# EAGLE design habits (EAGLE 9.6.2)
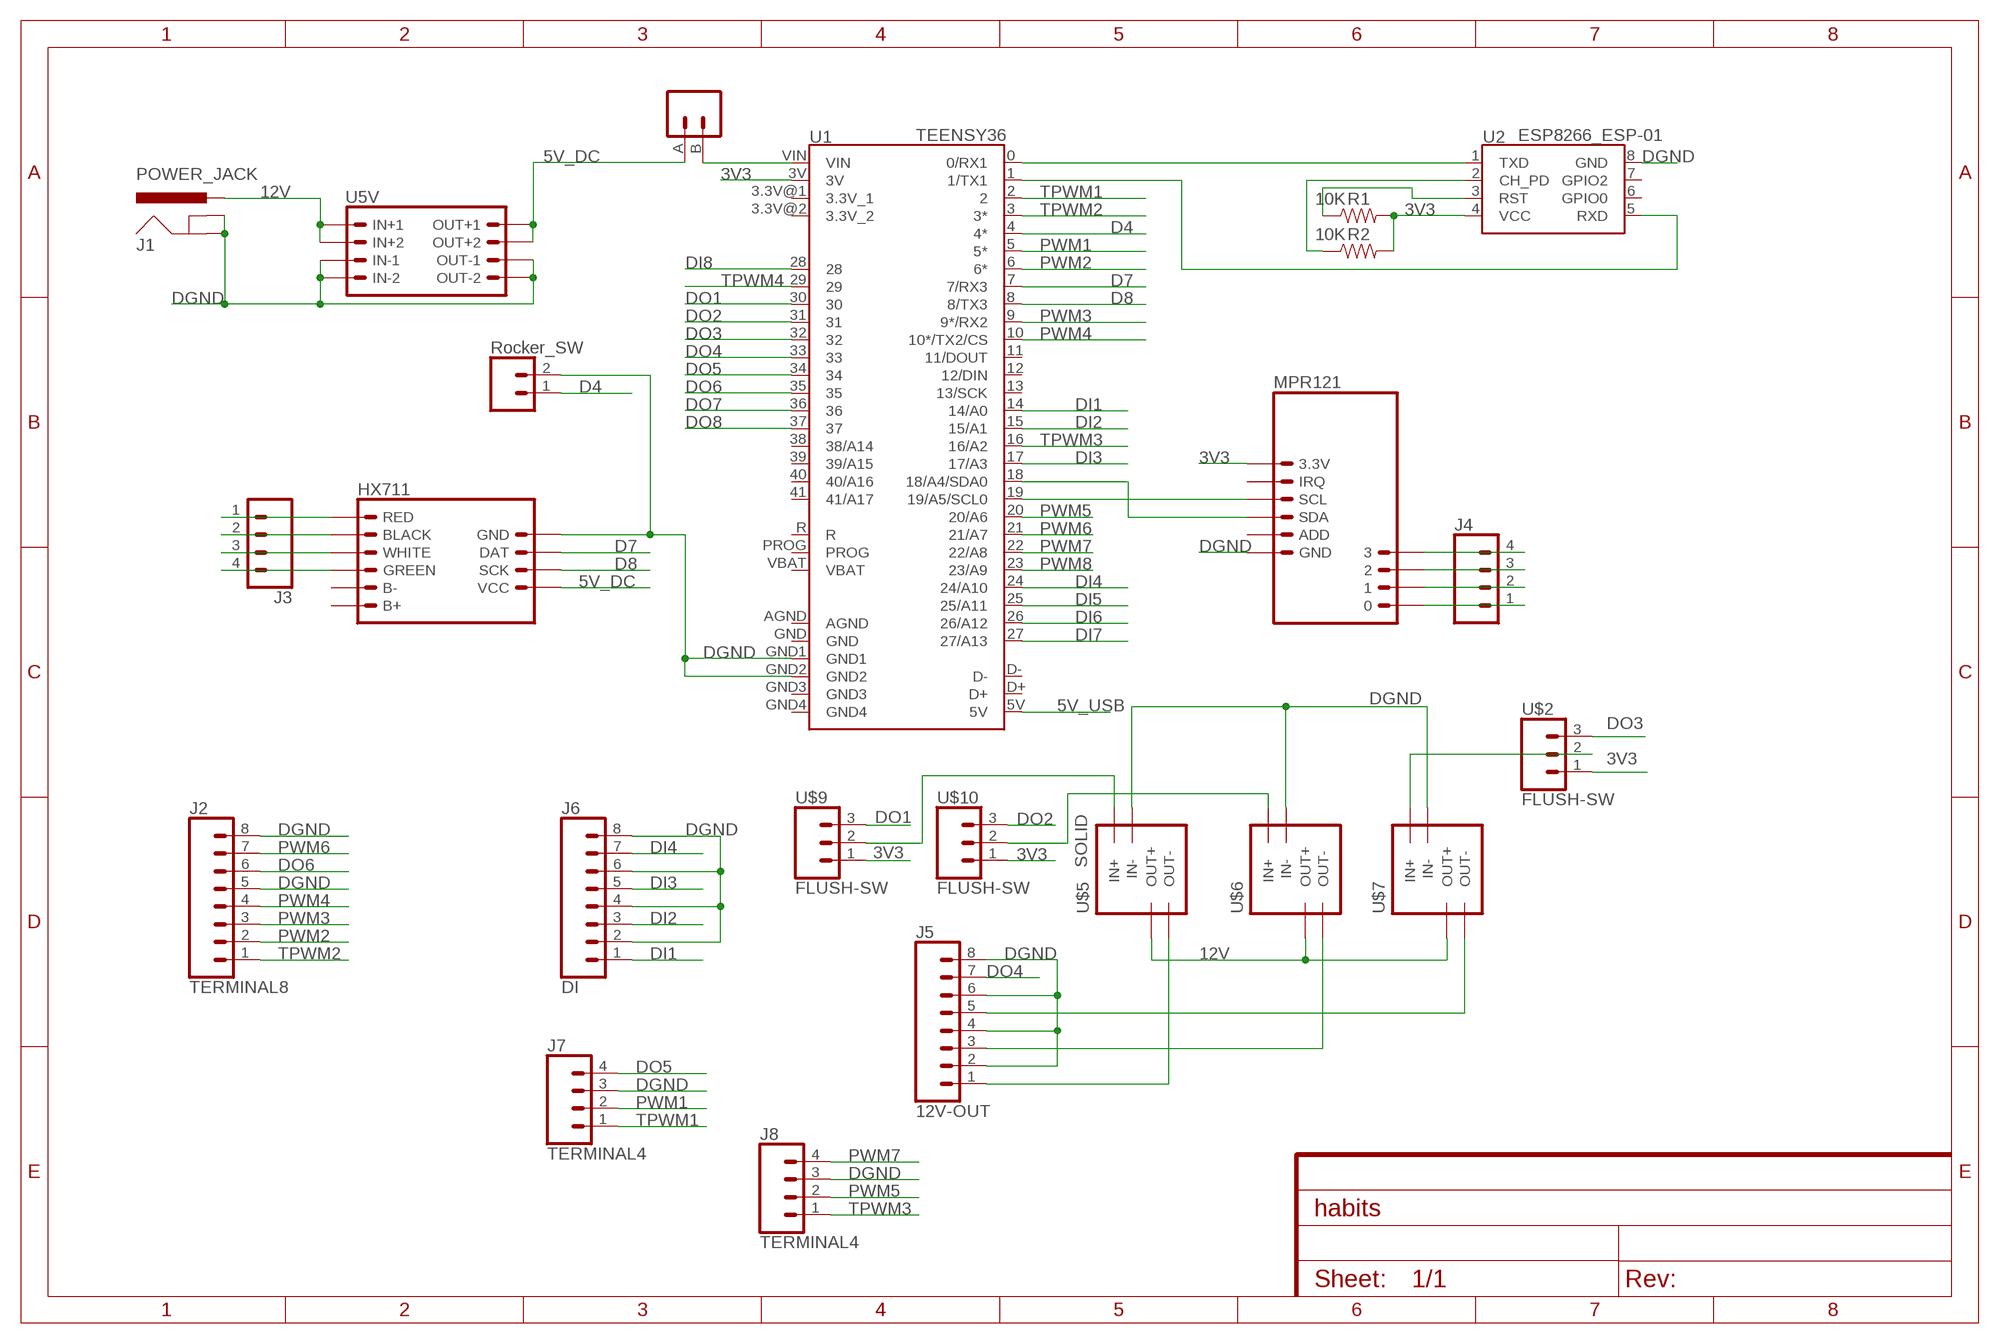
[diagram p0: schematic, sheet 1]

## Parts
J1  POWER_JACK  [POWER_JACK_PTH]
J2  TERMINAL8  [1X8]
J3  Load Cell  TERMINAL4  [1X4]
J4  LICKPORT  TERMINAL4  [1X4]
J5  12V-OUT  TERMINAL8  [1X8]
J6  DI  TERMINAL8  [1X8]
J7  TERMINAL4  [1X4]
J8  TERMINAL4  [1X4]
R1  10K  RESISTOR0603  [0603]
R2  10K  RESISTOR0603  [0603]
U1  TEENSY36  TEENSY_EXTENDEDW_SILK  [TEENSY_EXTENDED]
U2  ESP8266_ESP-01  [ESP8266_ESP-01]
U3  MPR121_4CH  [MPR121_4CH]
U5V  DC-DC-SMD  [DC-DC-SMD]
U$1  HX711  [HX711]
U$2  FLUSH-SW  [FLUSH-SW]
U$3  RESET_BUTTON  [RESET_BUTTON]
U$4  ROCKER-SW  [ROCKER-SW]
U$5  SOLID  [SOLID]
U$6  SOLID  [SOLID]
U$7  SOLID  [SOLID]
U$9  FLUSH-SW  [FLUSH-SW]
U$10  FLUSH-SW  [FLUSH-SW]

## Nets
3V3: R1.2 R2.2 U1.3V U2.4(VCC) U3.3.3V U$2.1 U$9.1 U$10.1
5V_DC: U5V.OUT+1 U5V.OUT+2 U$1.VCC U$3.A
5V_USB: U1.5V
12V: J1.PWR U5V.IN+1 U5V.IN+2 U$5.3(OUT+) U$6.3(OUT+) U$7.3(OUT+)
D4: U1.4(4*) U$4.1
D7: U1.7(7/RX3) U$1.DAT
D8: U1.8(8/TX3) U$1.SCL(SCK)
DGND: J1.GND J1.GNDBREAK J2.5 J2.8 J5.2 J5.4 J5.6 J5.8 J6.2 J6.4 J6.6 J6.8 J7.3 J8.3 U1.GND1 U1.GND2 U2.8(GND) U3.GND U5V.IN-1 U5V.IN-2 U5V.OUT-1 U5V.OUT-2 U$1.GND U$4.2 U$5.2(IN-) U$6.2(IN-) U$7.2(IN-)
DI1: J6.1 U1.14(14/A0)
DI2: J6.3 U1.15(15/A1)
DI3: J6.5 U1.17(17/A3)
DI4: J6.7 U1.24(24/A10)
DI5: U1.25(25/A11)
DI6: U1.26(26/A12)
DI7: U1.27(27/A13)
DI8: U1.28
DO1: U1.30 U$9.3
DO2: U1.31 U$10.3
DO3: U1.32 U$2.3
DO4: J5.7 U1.33
DO5: J7.4 U1.34
DO6: J2.6 U1.35
DO7: U1.36
DO8: U1.37
N$1: U1.0(0/RX1) U2.1(TXD)
N$2: U1.1(1/TX1) U2.5(RXD)
N$4: U1.VIN U$3.B
N$5: U1.18(18/A4/SDA0) U3.SDA
N$6: J5.1 U$5.4(OUT-)
N$7: U1.19(19/A5/SCL0) U3.SCL
N$8: J3.2 U$1.BLACK
N$9: J3.1 U$1.RED
N$10: J3.3 U$1.WHITE
N$11: J3.4 U$1.GREEN
N$12: J4.1 U3.0
N$13: J4.2 U3.1
N$14: J4.3 U3.2
N$15: J4.4 U3.3
N$16: J5.3 U$6.4(OUT-)
N$17: J5.5 U$7.4(OUT-)
N$19: R1.1 U2.3(RST)
N$20: U$5.1(IN+) U$9.2
N$21: U$6.1(IN+) U$10.2
N$22: R2.1 U2.2(CH_PD)
N$23: U$2.2 U$7.1(IN+)
PWM1: J7.2 U1.5(5*)
PWM2: J2.2 U1.6(6*)
PWM3: J2.3 U1.9(9*/RX2)
PWM4: J2.4 U1.10(10*/TX2/CS)
PWM5: J8.2 U1.20(20/A6)
PWM6: J2.7 U1.21(21/A7)
PWM7: J8.4 U1.22(22/A8)
PWM8: U1.23(23/A9)
TPWM1: J7.1 U1.2
TPWM2: J2.1 U1.3(3*)
TPWM3: J8.1 U1.16(16/A2)
TPWM4: U1.29
Unconnected: U1.11(11/DOUT) U1.12(12/DIN) U1.13(13/SCK) U1.38(38/A14) U1.39(39/A15) U1.40(40/A16) U1.41(41/A17) U1.GND4 U1.PROG U1.R U2.6(GPIO0) U2.7(GPIO2) U3.ADD U3.IRQ U$1.B+ U$1.B-

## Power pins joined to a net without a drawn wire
3.3V_1: U1.3.3V@1(3.3V_1)
3.3V_2: U1.3.3V@2(3.3V_2)
AGND: U1.AGND
D+: U1.D+
D-: U1.D-
GND: U1.GND
GND3: U1.GND3
VBAT: U1.VBAT

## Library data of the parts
J1 = SparkFun-Connectors:POWER_JACK: Power Jack Connector This is the standard 5.5mm barrel jack for power. The PTH is the most common, proven, reliable, footprint. The Slot footprint only works if the mill layer is transmitted to the PCB fab house so be warned. Here are the connectors we sell at SparkFun: DC Barrel Power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; PROD_ID: CONN-08197
J2 J5 J6 = habits:TERMINAL8
J3 J4 J7 J8 = habits:TERMINAL4
R1 R2 = SparkFun-Resistors:RESISTOR: Generic Resistor Package
U1 = SparkFun-Boards:TEENSY_EXTENDED: Teensy Footprint Extended Mechanical footprint with connectors for Teensy Development Board with ARM Cortex. SparkFun Products: Teensy 4.1 Teensy 3.6 Teensy 3.5 SparkFun Qwiic Shield for Teensy Extended Teensy Stackable Header Kit (Longer Version)
U2 = SparkFun-RF:ESP8266_ESP-01: ESP8266 ESP-01 Module The ESP8266 WiFi Module is a self contained SOC with integrated TCP/IP protocol stack that can give any microcontroller access to your WiFi network. The ESP8266 is capable of either hosting an application or offloading all Wi-Fi networking functions from another application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; SF_ID: WRL-13678
U3 = habits:MPR121_4CH
U5V = habits:DC-DC-SMD
U$1 = habits:HX711
U$2 U$9 U$10 = habits:FLUSH-SW
U$3 = habits:RESET_BUTTON
U$4 = habits:ROCKER-SW
U$5-U$7 = habits:SOLID

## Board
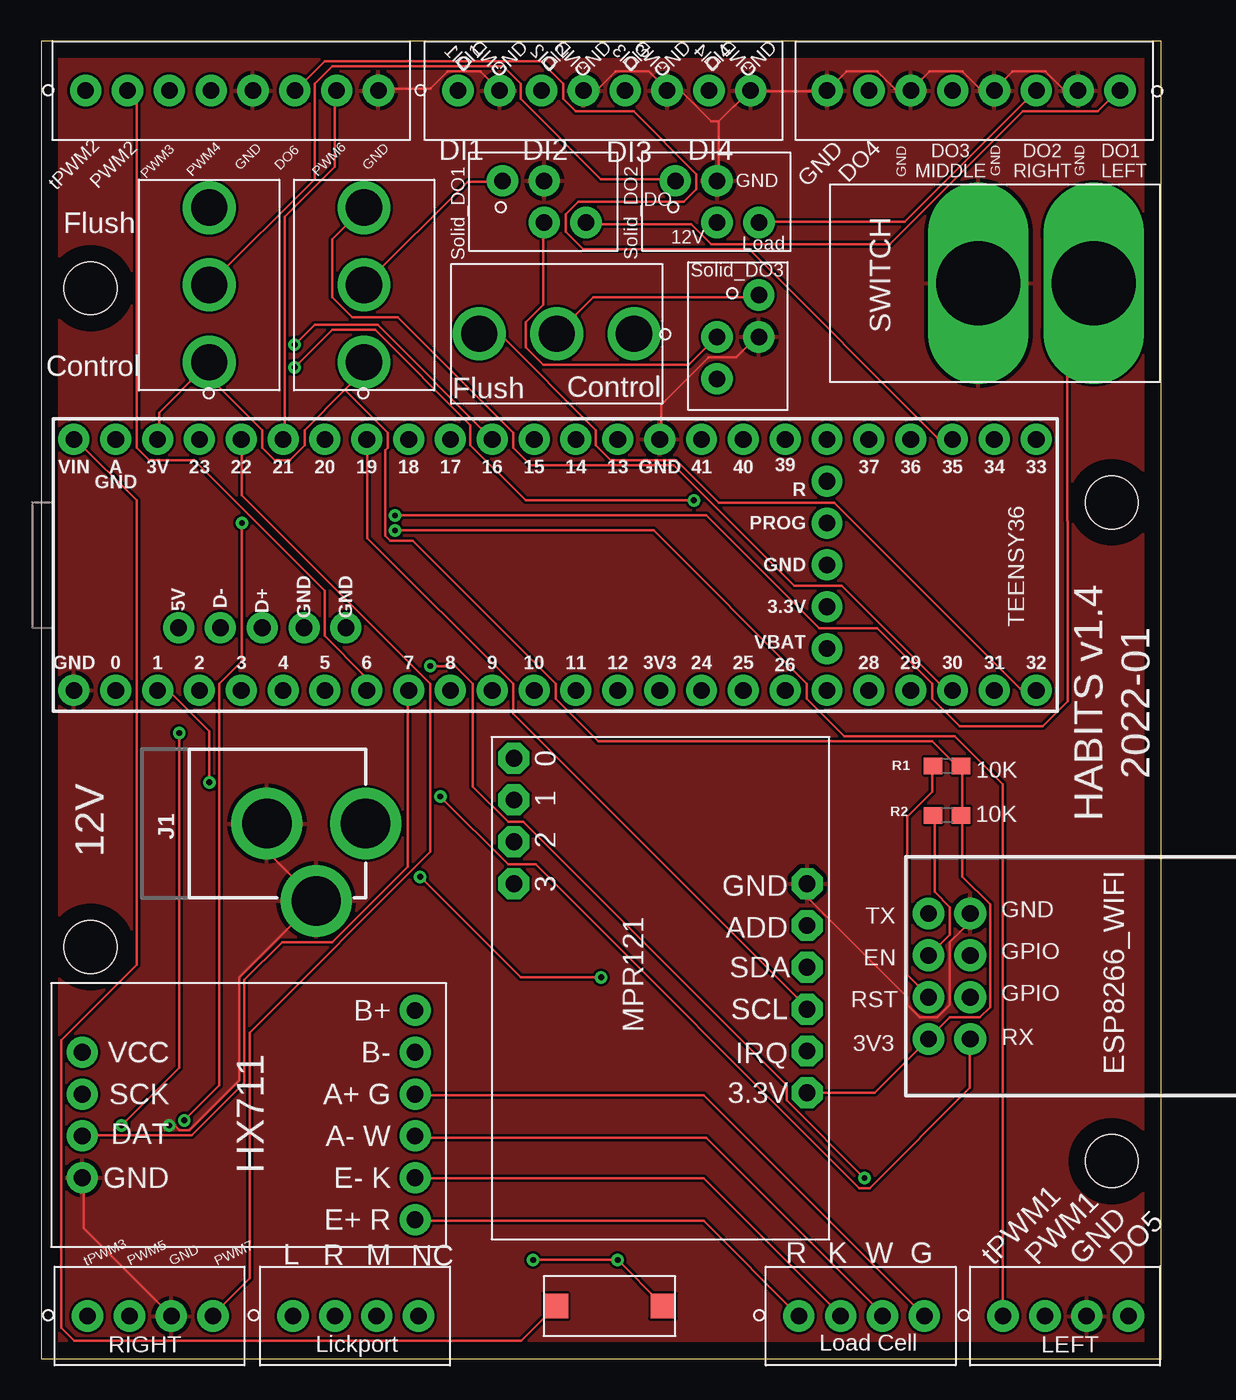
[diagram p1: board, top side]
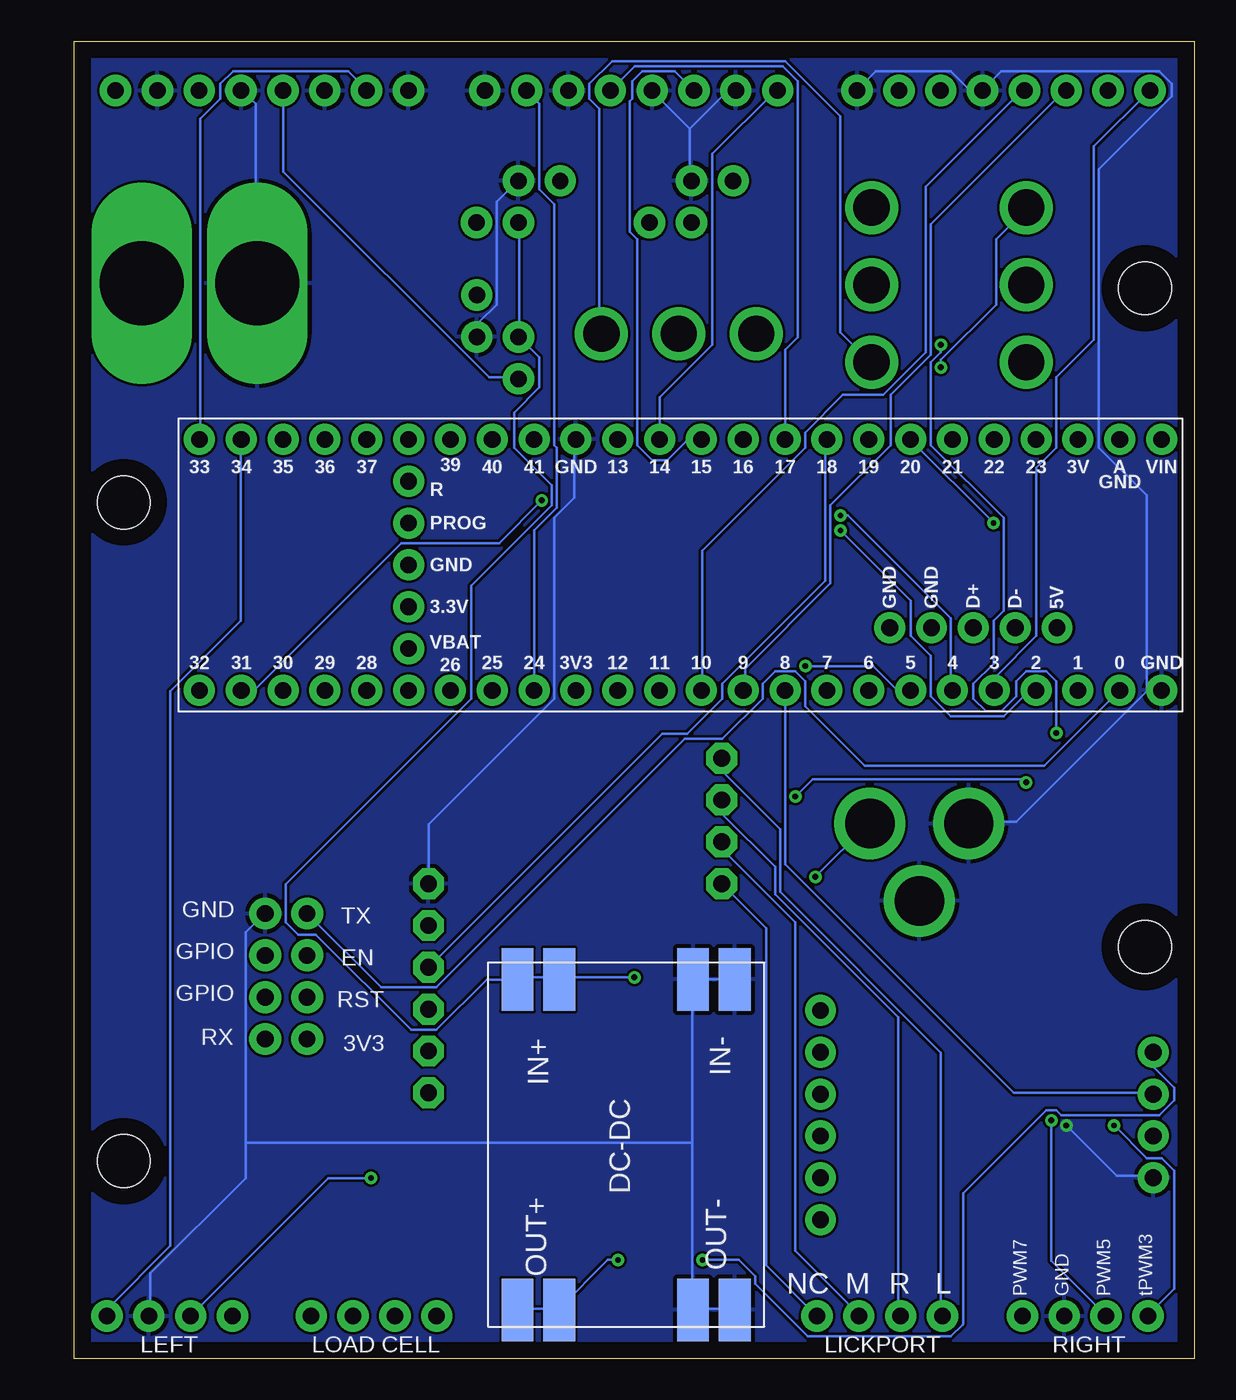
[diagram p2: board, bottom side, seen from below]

Size 68 x 80 mm. Coordinates in mm from the lower left corner, seen from the top.
Outline: 0,0 68,0 68,80 0,80 0,0
Copper layers (1*16): Top 0.035mm / dielectric 1.5mm / Bottom 0.035mm
Design rules "default": minimum track width 6mil, minimum drill 0.35mm, track to track 6mil, track to pad 6mil, pad to pad 6mil, via to via 6mil, smd to smd 6mil, copper to edge 40mil, drill to drill 6mil, minimum pad ring 10mil, minimum via ring 8mil, stop-mask expansion 4mil, vias tented up to drill 0mil, thermal gap 10mil
Holes 3.2 mm at 3,65 65,12 3,25 65,52

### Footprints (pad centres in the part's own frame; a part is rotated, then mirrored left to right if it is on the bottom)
POWER_JACK_PTH = drill 2.997 pad 4.318: GND 0,7.7; GNDBREAK 4.7,10.7; PWR 0,13.7
1X8 = drill 1 pad 1.9: 1 0,0; 2 2.54,0; 3 5.08,0; 4 7.62,0; 5 10.16,0; 6 12.7,0; 7 15.24,0; 8 17.78,0
1X4 = drill 1 pad 1.9: 1 0,0; 2 2.54,0; 3 5.08,0; 4 7.62,0
0603 = smd 1.1 x 1: 1 -0.85,0; 2 0.85,0
TEENSY_EXTENDED = drill 1.016 pad 1.88: 0 7.62,-13.97; 1 7.62,-11.43; 2 7.62,-8.89; 3 7.62,-6.35; 3.3V@1 7.62,19.05; 3.3V@2 2.54,29.21; 3V -7.62,-11.43; 4 7.62,-3.81; 5 7.62,-1.27; 5V 3.81,-10.16; 6 7.62,1.27; 7 7.62,3.81; 8 7.62,6.35; 9 7.62,8.89; 10 7.62,11.43; 11 7.62,13.97; 12 7.62,16.51; 13 -7.62,16.51; 14 -7.62,13.97; 15 -7.62,11.43; 16 -7.62,8.89; 17 -7.62,6.35; 18 -7.62,3.81; 19 -7.62,1.27; 20 -7.62,-1.27; 21 -7.62,-3.81; 22 -7.62,-6.35; 23 -7.62,-8.89; 24 7.62,21.59; 25 7.62,24.13; 26 7.62,26.67; 27 7.62,29.21; 28 7.62,31.75; 29 7.62,34.29; 30 7.62,36.83; 31 7.62,39.37; 32 7.62,41.91; 33 -7.62,41.91; 34 -7.62,39.37; 35 -7.62,36.83; 36 -7.62,34.29; 37 -7.62,31.75; 38 -7.62,29.21; 39 -7.62,26.67; 40 -7.62,24.13; 41 -7.62,21.59; AGND -7.62,-13.97; D+ 3.81,-5.08; D- 3.81,-7.62; GND 0,29.21; GND1 7.62,-16.51; GND2 -7.62,19.05; GND3 3.81,-2.54; GND4 3.81,0; PROG -2.54,29.21; R -5.08,29.21; VBAT 5.08,29.21; VIN -7.62,-16.51
ESP8266_ESP-01 = drill 1.016 pad 1.93: 1 -3.81,-11.13; 2 -1.27,-11.13; 3 1.27,-11.13; 4 3.81,-11.13; 5 3.81,-8.59; 6 1.27,-8.59; 7 -1.27,-8.59; 8 -3.81,-8.59
MPR121_4CH = drill 1.016 pad 1.88 octagon: 0 13.97,8.9; 1 11.43,8.9; 2 8.89,8.9; 3 6.35,8.9; 3.3V -6.35,-8.9; ADD 3.81,-8.9; GND 6.35,-8.9; IRQ -3.81,-8.9; SCL -1.27,-8.9; SDA 1.27,-8.9
DC-DC-SMD = smd 3.81 x 1.93: IN+1 -10.033,-4.065; IN+2 -10.033,-6.6; IN-1 -10.033,6.6; IN-2 -10.033,4.065; OUT+1 10.033,-4.065; OUT+2 10.033,-6.6; OUT-1 10.033,6.6; OUT-2 10.033,4.065
HX711 = drill 1.016 pad 1.88: B+ 6.35,-10.1; B- 3.81,-10.1; BLACK -3.81,-10.1; DAT -1.27,10.1; GND -3.81,10.1; GREEN 1.27,-10.1; RED -6.35,-10.1; SCL 1.27,10.1; VCC 3.81,10.1; WHITE -1.27,-10.1
FLUSH-SW = drill 2.2 pad 3: 1 0,0; 2 4.7,0; 3 9.4,0
RESET_BUTTON = smd 1.5 x 1.5: A -3.25,0; B 3.25,0
ROCKER-SW = drill 5.1 pad 6.1 long: 1 0,0; 2 7,0
SOLID = drill 1 pad 1.9: 1 0,0; 2 2.54,0; 3 2.54,-2.54; 4 5.08,-2.54

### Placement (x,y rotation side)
J1  6,32.5 270 top
J2  2.7,77 0 top
J3  46,2.6 0 top
J4  15.29,2.6 0 top
J5  65.5,77 180 top
J6  25.3,77 0 top
J7  58.4,2.6 0 top
J8  2.82,2.6 0 top
R1  55,36 0 top
R2  55,33 0 top
U1  18.5,48.2 270 top
U2  65,23.23 270 top
U3  37.6,22.5 90 top
U5V  34.5,13 270 bottom
U$1  12.6,14.8 90 top
U$2  36,62.23 180 top
U$3  34.5,3.2 180 top
U$4  63.9,65.3 180 top
U$5  28,71.52 0 top
U$6  38.5,71.52 0 top
U$7  43.57,64.58 270 top
U$9  19.6,60.5 90 top
U$10  10.2,60.5 90 top

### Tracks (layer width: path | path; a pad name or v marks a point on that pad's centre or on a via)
3V3
  Top 0.152: U3.3.3V 46.63,16.15 50.6,16.15 53.8,19.36 U2.4 53.95,19.51 55.17,20.73 57,20.73 57.61,21.34 57.61,27.58 55.93,29.26 55.93,32.92 R2.2 55.93,33.07 55.93,35.97 R1.2 55.78,36.12 55.47,36.12 54.1,37.49 33.83,37.49 31.24,40.08 31.24,41 22.55,49.68 21.18,49.68 20.88,49.99 20.88,55.17 21.03,55.32 21.03,56.24 18.44,58.83 | 9.75,60.05 10.06,60.35 U$10.1 9.75,60.05 | 9.75,60.05 7.16,57.45 7.16,55.93 U1.3V | 18.44,58.83 16,56.39 16,55.47 15.09,54.56 14.17,54.56 13.41,55.32 13.41,56.39 9.75,60.05 | 18.44,58.83 19.51,59.89 19.51,60.35 U$9.1
  Bottom 0.152: U$2.1 36.12,62.33 36.12,75.89 36.73,76.5 36.73,77.42 35.36,78.79 24.84,78.79 21.49,75.44 21.49,62.33 19.66,60.5 U$9.1
5V_DC  (via drill 0.35)
  Top 0.152: U$3.A 37.64,3.05 37.64,3.36 v35,6 v29.87,6
  Bottom 0.152: U$1.VCC 2.44,18.59 2.44,17.68 1.22,16.46 1.22,15.7 2.13,14.78 8.08,14.78 8.38,15.09 8.99,15.09 14.02,10.06 14.02,2.13 14.08,2.08 14.78,1.37 23.47,1.37 26.67,4.57 26.67,5 27.67,6 v29.87,6 | U5V.OUT+2 41,3.05 38.71,3.05 U5V.OUT+1 38.56,3.05 35.6,6 v35,6
12V  (via drill 0.35)
  Top 0.152: U$5.3 30.48,68.89 30.48,64.01 29.41,62.94 29.41,61.42 30.48,60.35 39.32,60.35 41,62.03 U$7.3 | v23.01,29.26 29.11,23.16 v34,23.16
  Bottom 0.152: U$6.3 41,68.89 41,62.18 U$7.3 41,62.03 39.78,60.81 39.78,58.98 41.3,57.45 41.3,55.32 39.01,53.03 39.01,51.82 43.89,46.94 43.89,40.08 55.17,28.8 55.17,26.52 54.41,25.76 53.34,25.76 47.55,19.96 46.02,19.96 42.98,23.01 41.15,23.01 U5V.IN+2 41,23.16 38.71,23.16 U5V.IN+1 38.56,23.16 v34,23.16 | v23.01,29.26 19.81,32.46 J1.PWR
D4  (via drill 0.35)
  Top 0.152: v21.49,51.21 40.39,51.21 47.24,44.35 50.75,44.35 54.1,41 54.1,40.08 55.78,38.41 60.81,38.41 62.33,39.93 62.33,50.86 62.31,50.88 62.31,63.68 63.86,65.23 U$4.1
  Bottom 0.152: v21.49,51.21 21.03,51.21 14.78,44.96 14.78,40.69 U1.4
D7
  Top 0.152: U$1.DAT 2.59,13.56 9.14,13.56 12.34,16.76 12.34,23.01 14.63,25.3 17.68,25.3 22.25,29.87 22.25,40.54 U1.7
D8
  Bottom 0.152: U$1.SCL 2.59,16.15 10.97,16.15 24.84,30.02 24.84,40.54 U1.8
DGND  (via drill 0.35)
  Top 0.152: U3.GND 46.63,28.8 46.63,27.89 52.58,21.95 52.58,21.49 53.34,20.73 54.41,20.73 55.17,21.49 55.17,25.3 56.39,26.52 56.39,26.98 U2.8 | U$1.GND 2.59,10.97 2.59,7.92 7.77,2.74 J8.3 | v7.77,14.17 8.08,14.17 8.38,13.87 8.99,13.87 12.04,16.92 12.04,23.16 16.61,27.74 J1.GNDBREAK 16.61,27.89 13.72,30.79 13.72,32.46 J1.GND | J2.8 20.57,77.11 23.62,77.11 24.69,78.18 26.67,78.18 27.74,77.11 J6.2 | U1.GND2 37.64,55.93 37.64,57.91 40.54,60.81 42.22,60.81 43.43,62.03 U$7.2 | 41.15,75.13 41.15,71.63 U$6.2 | 41.15,75.13 42.98,76.96 J6.8 43.13,76.96 47.7,76.96 J5.8 47.85,77.11 48.92,78.18 50.75,78.18 51.82,77.11 52.73,77.11 J5.6 52.88,77.11 53.95,78.18 55.93,78.18 57,77.11 57.76,77.11 J5.4 57.91,77.11 58.98,78.18 60.96,78.18 62.03,77.11 62.94,77.11 J5.2 | 41.15,75.13 40.69,75.13 38.86,76.96 38.1,76.96 J6.6 37.95,77.11 36.88,78.18 34.9,78.18 33.83,77.11 33.07,77.11 J6.4
  Bottom 0.152: U5V.OUT-1 28.04,3.05 30.33,3.05 U5V.OUT-2 30.48,3.05 30.48,13.11 | 30.48,23 30.48,23.01 U5V.IN-2 | 30.48,23 30.48,13.11 | 57.61,13.11 57.61,25.91 56.54,26.98 U2.8 | 57.61,13.11 57.61,10.97 63.4,5.18 63.4,2.74 J7.3 | 57.61,13.11 30.48,13.11 | 2.9,40.54 2.13,40.54 U1.GND1 2.9,40.54 | 2.9,40.54 10.82,32.61 13.56,32.61 J1.GND | v7.77,14.17 4.72,11.12 2.59,11.12 U$1.GND | J2.8 20.42,77.11 19.36,78.18 14.78,78.18 13.72,77.11 12.95,77.11 J2.5 12.8,77.11 11.73,78.18 2.13,78.18 1.37,77.42 1.37,76.66 5.79,72.24 5.79,55.32 2.9,52.43 2.9,40.54 | 30.63,74.68 30.63,71.63 U$5.2 | 30.63,74.68 32.92,76.96 J6.4 | 30.63,74.68 28.35,76.96 27.89,76.96 J6.2 | U$7.2 43.43,62.18 43.43,62.94 42.37,64.01 42.37,70.26 41.15,71.48 U$6.2 | U$4.2 57,65.38 57,76.2 57.76,76.96 J5.4 | U3.GND 46.48,28.96 46.48,32.46 38.86,40.08 38.86,51.05 37.64,52.27 37.64,55.78 U1.GND2 | U5V.IN-2 30.45,23.03 30.48,23 | U5V.IN-1 U5V.IN-2
  pour Top: 0,0 68,0 68,80 0,80
  pour Bottom: 0,0 68,0 68,80 0,80
DI1
  Bottom 0.152: U1.14 32.46,55.93 32.46,58.37 29.26,61.57 29.26,73.15 25.45,76.96 J6.1
DI2
  Bottom 0.152: U1.15 30.02,55.78 30.79,55.78 32,54.56 32.92,54.56 33.83,55.47 33.83,67.97 34.29,68.43 34.29,76.35 34.14,76.5 34.14,77.57 33.53,78.18 31.55,78.18 30.48,77.11 J6.3
DI3
  Bottom 0.152: U1.17 24.84,55.93 24.84,61.27 24.08,62.03 24.08,77.57 24.99,78.49 33.98,78.49 35.36,77.11 J6.5
DI4
  Bottom 0.152: U1.24 40.08,40.69 40.08,50.29 38.71,51.66 38.71,55.32 38.86,55.47 38.86,70.1 39.78,71.02 39.78,76.2 40.54,76.96 J6.7
DO1
  Top 0.152: U1.30 55.32,40.69 54.86,40.69 48.62,46.94 45.72,46.94 38.41,54.25 29.72,54.25 28.65,55.32 28.65,56.24 21.64,63.25 18.9,63.25 17.68,64.47 17.68,67.97 19.51,69.8 U$9.3
DO2  (via drill 0.35)
  Top 0.152: v39.62,52.12 29.41,52.12 26.06,55.47 26.06,56.69 20.27,62.48 17.68,62.48 v15.39,60.2
  Bottom 0.152: v39.62,52.12 42.22,49.53 48.16,49.53 57,40.69 57.76,40.69 U1.31 | v15.39,60.2 15.39,60.66 12.04,64.01 12.04,67.97 10.21,69.8 U$10.3
DO3
  Top 0.152: U1.32 60.35,40.69 59.44,40.69 48.16,51.97 41.15,51.97 38.56,54.56 34.59,54.56 33.68,55.47 33.68,56.39 27.89,62.18 26.67,62.18 U$2.3
DO4
  Bottom 0.152: U1.33 60.35,55.93 60.35,75.29 59.13,76.5 59.13,77.42 58.37,78.18 51.36,78.18 50.29,77.11 J5.7
DO5
  Bottom 0.152: U1.34 57.91,55.78 57.91,44.81 62.18,40.54 62.18,6.86 65.99,3.05 65.99,2.74 J7.4
DO6
  Top 0.152: U1.35 55.32,55.93 54.41,55.93 42.98,67.36 32.92,67.36 31.85,68.43 31.85,69.49 32.61,70.26 39.01,70.26 39.78,71.02 39.78,71.93 35.97,75.74 32.46,75.74 31.7,76.5 31.7,77.42 30.33,78.79 17.22,78.79 15.54,77.11 J2.6
N$1
  Bottom 0.152: U2.1 53.8,26.98 49.38,22.55 46.02,22.55 30.94,37.64 28.65,37.64 26.21,40.08 26.21,41 25.45,41.76 24.23,41.76 23.62,41.15 23.62,39.62 20,36 9.11,36 U1.0
N$2  (via drill 0.35)
  Top 0.152: v10.21,35 10.21,38.1 7.77,40.54 7.16,40.54 U1.1 | v24.23,34.14 28.35,30.02 30.02,30.02 49.68,10.36 50.29,10.36 56.39,16.46 56.39,19.36 U2.5
  Bottom 0.152: v24.23,34.14 23.18,35.19 10.39,35.19 v10.21,35
N$4
  Top 0.152: U1.VIN 2.13,55.78 5.79,52.12 5.79,23.93 1.22,19.36 1.22,1.87 2,1.09 29.14,1.09 U$3.B
N$5
  Bottom 0.152: U1.18 22.4,55.78 22.4,47.24 28.65,41 28.65,40.08 30.79,37.95 32.31,37.95 46.48,23.77 U3.SDA
N$6
  Top 0.152: U$5.4 33.22,68.89 39.47,68.89 40.69,67.67 51.51,67.67 59.59,75.74 64.16,75.74 65.38,76.96 J5.1
N$7
  Top 0.152: U1.19 19.81,55.78 19.81,49.84 28.65,41 28.65,39.17 46.48,21.34 U3.SCL
N$8
  Top 0.152: U$1.BLACK 22.71,10.97 40.23,10.97 48.46,2.74 J3.2
N$9
  Top 0.152: U$1.RED 22.71,8.38 40.22,8.38 J3.1
N$10
  Top 0.152: U$1.WHITE 22.71,13.41 40.39,13.41 51.05,2.74 J3.3
N$11
  Top 0.152: U$1.GREEN 22.71,16 40.23,16 53.49,2.74 J3.4
N$12
  Bottom 0.152: U3.0 28.65,36.42 28.65,35.66 25.15,32.16 25.15,28.35 15.39,18.59 15.39,2.74 J4.1
N$13
  Bottom 0.152: U3.1 28.65,33.83 28.65,33.07 25.45,29.87 25.45,28.19 17.98,20.73 17.98,2.74 J4.2
N$14
  Bottom 0.152: U3.2 28.65,31.24 28.65,30.94 24.23,26.52 24.23,6.55 20.42,2.74 J4.3
N$15
  Bottom 0.152: J4.4 26,5.69 26,26.15 U3.3
N$16
  Top 0.152: U$6.4 43.59,69.04 52.43,69.04 60.35,76.96 J5.3
N$17
  Bottom 0.152: U$7.4 41.15,59.59 42.82,59.59 55.32,72.08 55.32,76.96 J5.5
N$19
  Top 0.152: R1.1 54.1,35.97 54.1,34.44 52.58,32.92 52.58,23.32 53.8,22.1 U2.3
N$20
  Top 0.152: U$5.1 27.89,71.48 25.91,71.48 19.66,65.23 U$9.2
N$21
  Top 0.152: U$6.1 38.41,71.63 33.98,71.63 29.11,76.5 29.11,77.42 28.04,78.49 17.68,78.49 16.61,77.42 16.61,71.63 10.21,65.23 U$10.2
N$22
  Top 0.152: R2.1 54.25,32.92 54.25,28.35 55.17,27.43 55.17,25.76 53.95,24.54 U2.2
N$23
  Top 0.152: U$7.1 43.43,64.47 33.53,64.47 31.39,62.33 U$2.2
PWM1  (via drill 0.35)
  Top 0.152: v23.62,42.06 25.15,42.06 26.21,41 26.21,34.75 28.35,32.61 29.26,32.61 45.26,16.61 45.26,15.7 v49.99,10.97
  Bottom 0.152: v23.62,42.06 19.51,42.06 18.14,40.69 17.37,40.69 U1.5 | v49.99,10.97 52.58,10.97 60.81,2.74 J7.2
PWM2
  Top 0.152: U1.6 19.66,40.69 19.66,41.45 17.22,43.89 17.22,46.63 9.3,54.56 6.55,54.56 5.79,55.32 5.79,76.5 5.33,76.96 J2.2
PWM3
  Bottom 0.152: U1.9 27.28,40.69 27.28,41.91 22.1,47.09 22.1,51.82 18.44,55.47 18.44,58.52 16,60.96 16,68.89 7.92,76.96 J2.3
PWM4
  Bottom 0.152: U1.10 29.87,40.69 29.87,49.07 23.62,55.32 23.62,56.24 21.34,58.52 18.9,58.52 16.31,61.11 16.31,71.17 10.36,77.11 J2.4
PWM5  (via drill 0.35)
  Top 0.152: v12.19,50.75 12.19,42.37 10.82,41 10.82,16.61 v8.69,14.48
  Bottom 0.152: v12.19,50.75 17.22,55.78 U1.20 | v8.69,14.48 8.69,5.94 5.49,2.74 J8.2
PWM6
  Top 0.152: U1.21 14.78,55.93 14.78,69.34 17.83,72.39 17.83,76.96 J2.7
PWM7
  Top 0.152: U1.22 12.19,55.78 12.19,52.43 23.62,41 23.62,30.79 12.65,19.81 12.65,4.88 10.52,2.74 J8.4
TPWM1  (via drill 0.35)
  Top 0.152: v21.49,50.29 37.19,50.29 46.48,41 46.48,40.08 48.77,37.8 55.47,37.8 58.37,34.9 58.37,2.74 J7.1
  Bottom 0.152: v21.49,50.29 17.22,46.02 17.22,43.89 16,42.67 16,40.23 14.78,39.01 11.58,39.01 10.06,40.54 9.75,40.54 U1.2
TPWM2
  Bottom 0.152: U1.3 12.04,40.69 12.04,41.45 9.6,43.89 9.6,54.1 8.38,55.32 8.38,59.59 6.1,61.87 6.1,73.61 2.74,76.96 J2.1
TPWM3  (via drill 0.35)
  Top 0.152: v15.39,61.57 16.61,62.79 20.42,62.79 27.28,55.93 U1.16 | v8.38,38 8.38,17.68 v4.88,14.17
  Bottom 0.152: v15.39,61.57 15.39,61.11 16,60.5 16,55.47 11.58,51.05 11.58,45.41 12.19,44.81 12.19,42.22 13.41,41 13.41,40.08 12.65,39.32 11.73,39.32 10.82,40.23 10.82,41.15 10.21,41.76 8.99,41.76 8.38,41.15 v8.38,38 | v4.88,14.17 2.9,12.19 1.98,12.19 1.22,11.43 1.22,4.27 2.74,2.74 J8.1

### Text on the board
tPlace: DI1 | DI1 | GND | GND | DI2 | DI2 | GND | GND | DI3 | DI3 | GND | GND | DI4 | DI4 | GND | GND | DI1 | DI2 | DI3 | DI4 | DO3 / MIDDLE | DO2 / RIGHT | PWM3 | PWM4 | GND | DO6 | PWM6 | GND | GND | GND | GND | DO1 / LEFT | tPWM2 | PWM2 | GND | GND | DO4 | Flush | DO | 12V | Solid_DO1 | Solid_DO2 | Load | Solid_DO3 | Control | Flush | Control | TEENSY36 | HABITS v1.4 / 2022-01 | 12V | GND | TX | EN | GPIO | GPIO | RST | 3V3 | RX | ESP8266_WIFI | L | R | M | tPWM3 | PWM5 | GND | PWM7 | NC | R | K | W | G | tPWM1 | PWM1 | GND | DO5 | RIGHT | LEFT
bPlace: GND | TX | EN | GPIO | GPIO | RST | 3V3 | RX | tPWM3 | PWM5 | GND | PWM7 | L | R | M | NC | RIGHT | LICKPORT | LOAD CELL | LEFT

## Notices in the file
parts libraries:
SparkFun-Boards: Licensing: Creative Commons ShareAlike 4.0 International - https://creativecommons.org/licenses/by-sa/4.0
